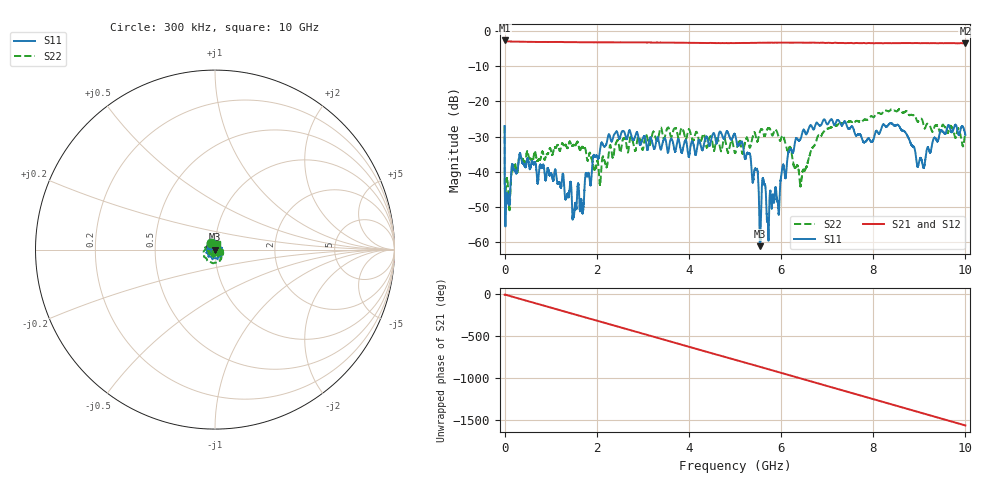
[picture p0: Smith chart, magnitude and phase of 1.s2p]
!Keysight Technologies,N5232A,MY52221221,A.10.65.11
!Date: Thursday, May 09, 2024 19:59:05
!Correction: S11(Full 2 Port(1,4))
!S41(Full 2 Port(1,4))
!S14(Full 2 Port(1,4))
!S44(Full 2 Port(1,4))
!S2P File: Measurements: S11, S41, S14, S44:
# Hz S  RI  R 50
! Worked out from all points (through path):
!   16001 points, 300 kHz to 10 GHz, reference 50 ohm
!   highest |S21| = -2.67 dB at 300 kHz (marker M1); lowest = -3.5 dB at 10 GHz (marker M2)
!   group delay of S21, straight-line fit = 436 ps
!   lowest |S11| = -61.1 dB at 5.54 GHz (marker M3), VSWR 1.00, Z = 49.9 - j0.0614 ohm
!   |S11| at or under -10 dB: start of sweep to end of sweep
!   |S22| runs from -50.9 to -22.2 dB; largest |S21 - S12| = 0.017
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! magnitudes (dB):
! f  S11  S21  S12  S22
! 300 kHz  -27.0  -2.7  -2.6  -27.0
! 57.17 MHz  -46.1  -2.9  -2.9  -41.9
! 177.2 MHz  -38.1  -3.0  -3.0  -39.4
! 349.7 MHz  -35.3  -3.0  -3.0  -35.9
! 1.667 GHz  -48.2  -3.2  -3.2  -33.1
! 2.06 GHz  -34.9  -3.2  -3.2  -42.6
! 2.256 GHz  -29.4  -3.2  -3.2  -35.1
! 3.334 GHz  -30.5  -3.3  -3.3  -30.4
! 5 GHz  -29.4  -3.4  -3.4  -34.6
! 5.461 GHz  -39.2  -3.3  -3.3  -30.6
! 5.54 GHz  -61.1  -3.3  -3.3  -28.6
! 5.623 GHz  -42.8  -3.3  -3.3  -29.3
! 5.71 GHz  -53.4  -3.3  -3.3  -27.7
! 5.938 GHz  -50.1  -3.3  -3.3  -29.7
! 6.179 GHz  -34.0  -3.3  -3.3  -33.1
! 6.427 GHz  -30.5  -3.3  -3.3  -43.8
! 6.667 GHz  -27.1  -3.3  -3.3  -33.4
! 7.816 GHz  -31.5  -3.4  -3.4  -25.1
! 8.334 GHz  -26.6  -3.4  -3.4  -22.8
! 9.083 GHz  -38.6  -3.4  -3.4  -26.1
! 9.48 GHz  -28.1  -3.4  -3.4  -27.7
! 10 GHz  -29.5  -3.5  -3.5  -28.9
